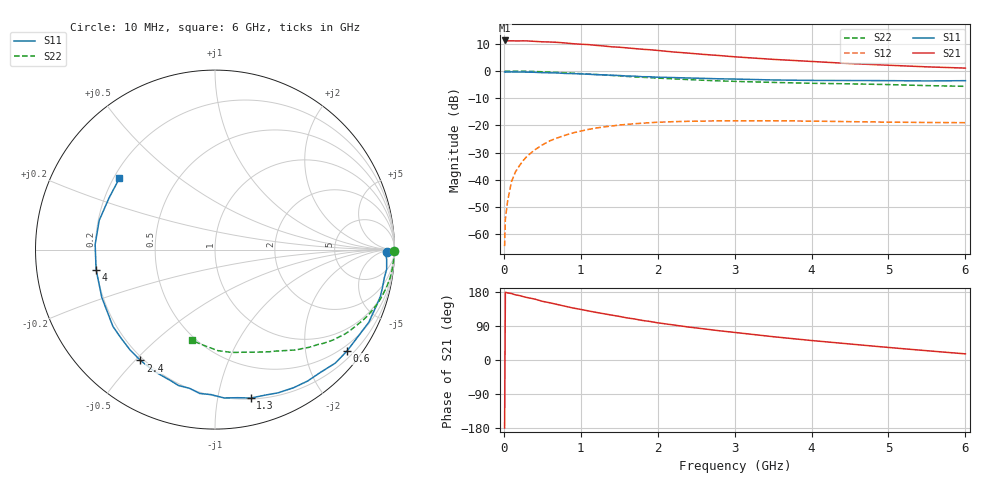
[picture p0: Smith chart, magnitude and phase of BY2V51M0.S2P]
! SIEMENS Small Signal Semiconductors
! BFY420
! Si NPN RF SIEGET Grounded Emitter Transistor in MICRO-X
! VCE = 2.5 V  IC = 1 mA
! Common Emitter S-Parameters:  October  1996
# GHz  S  MA  R  50
!  f  S11  S21  S12  S22
! GHz  MAG  ANG  MAG  ANG  MAG  ANG  MAG  ANG
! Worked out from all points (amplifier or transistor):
!   36 points, 10 MHz to 6 GHz, reference 50 ohm
!   highest |S21| = 11.2 dB at 10 MHz (marker M1)
!   |S21| within 3 dB of that: start of sweep to 1.708 GHz
!   unconditionally stable (mu >= 1): 4.54 GHz to end of sweep
!   at 250 MHz: K = 0.04, MSG = 22.1 dB, |S12| = -33.0 dB
!   at 1.4 GHz: K = 0.20, MSG = 14.6 dB, |S12| = -20.2 dB
!   at 6 GHz: K = 1.34, MAG = 6.5 dB, |S12| = -19.0 dB
!   S11 on the Smith chart (normalised r, x): 10 MHz: 43, -15; 600 MHz: 0.36, -2.91; 1.3 GHz: 0.21, -1.25; 2.4 GHz: 0.19, -0.52; 4 GHz: 0.20, -0.08; 6 GHz: 0.22, +0.32
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0.01  0.9595 -0.8  3.649 -179.5  0.0006 92.7  0.9987 -0.3
0.02  0.9523 -1.3  3.644 178.8  0.0019 85.7  0.9955 -0.6
0.05  0.958 -3.3  3.588 177.0  0.0041 86.5  0.9972 -1.5
0.1  0.9628 -6.5  3.594 175.4  0.0093 86.4  0.9974 -3.1
0.15  0.9563 -9.5  3.582 171.9  0.0139 83.0  0.9945 -4.6
0.3  0.9526 -18.9  3.581 164.9  0.0269 79.0  0.9885 -9.1
0.4  0.9478 -25.3  3.511 160.9  0.0353 75.1  0.9793 -12.1
0.5  0.9325 -31.3  3.445 154.9  0.0437 71.0  0.9685 -15.0
0.6  0.9276 -37.5  3.418 150.9  0.0521 67.5  0.9573 -17.8
0.8  0.9016 -49.4  3.278 141.7  0.0661 59.9  0.9272 -23.4
1.1  0.872 -66.2  3.061 129.5  0.0844 50.7  0.8786 -30.7
1.3  0.8506 -76.5  2.886 122.1  0.0938 44.6  0.8457 -35.1
1.6  0.808 -91.6  2.663 111.1  0.1045 36.7  0.796 -41.1
1.8  0.7856 -100.4  2.515 104.4  0.1096 32.3  0.7675 -44.4
2.2  0.7581 -116.6  2.243 92.6  0.117 24.2  0.7192 -51.0
2.4  0.7442 -123.9  2.134 87.0  0.1188 21.0  0.6949 -53.9
2.8  0.7188 -137.0  1.927 77.2  0.1211 15.1  0.6579 -59.3
3.5  0.6847 -157.1  1.639 61.5  0.1216 7.8  0.617 -67.8
4  0.6719 -170.4  1.5 51.4  0.1198 4.1  0.5947 -74.0
4.5  0.6683 177.5  1.371 42.2  0.1171 1.1  0.581 -80.6
5.5  0.6568 154.1  1.193 24.5  0.113 -0.7  0.5393 -95.8
6  0.6646 143.2  1.132 16.2  0.1122 -0.1  0.5225 -104.3
